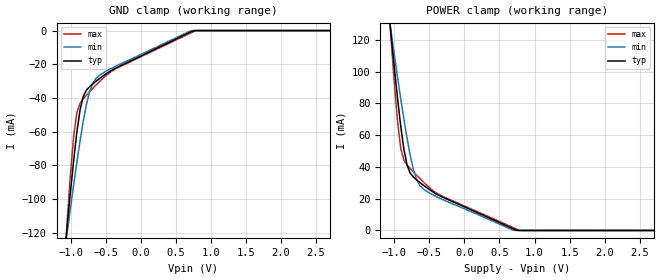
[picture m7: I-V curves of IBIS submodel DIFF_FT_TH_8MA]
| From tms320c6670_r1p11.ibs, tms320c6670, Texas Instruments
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|   Model Cell DIFF_FT_TH_8MA
|DIFF_FT_TH_8MA
[Submodel]   DIFF_FT_TH_8MA
Submodel_type   Dynamic_clamp
[POWER_clamp]
|   voltage   I(typ)   I(min)   I(max)
-1.5V     342.3mA    275.7mA    437.3mA
-1.091V   143.7mA    139.6mA    149.7mA
-1.046V   122.9mA    125.1mA    120.4mA
-954.6mV  83.55mA    96.8mA     69mA
-909.2mV  65.98mA    83.23mA    51.97mA
-818.2mV  41.15mA    58.15mA    41.18mA
-727.3mV  33.6mA     38.36mA    36.86mA
-636.4mV  30.26mA    28.37mA    32.77mA
-545.5mV  27.22mA    24.85mA    28.87mA
-318.2mV  21.1mA     19.57mA    21.61mA
772.8mV   0A         0A         294.7uA
3V        0A         0A         0A
[GND_clamp]
|   voltage   I(typ)   I(min)   I(max)
-1.5V     -334.4mA   -269.8mA   -427.4mA
-1.091V   -135.7mA   -133.7mA   -140mA
-1.046V   -115.1mA   -119.3mA   -111.2mA
-954.6mV  -76.62mA   -91.21mA   -62.46mA
-909.2mV  -60.01mA   -77.87mA   -48.55mA
-863.7mV  -46.93mA   -65.23mA   -43.02mA
-818.2mV  -38.98mA   -53.64mA   -40.41mA
-727.3mV  -33.23mA   -36mA      -36.22mA
-636.4mV  -30.06mA   -28.37mA   -32.26mA
-545.5mV  -27.17mA   -25.39mA   -28.56mA
772.8mV   0A         0A         -285.7uA
3V        0A         0A         0A
